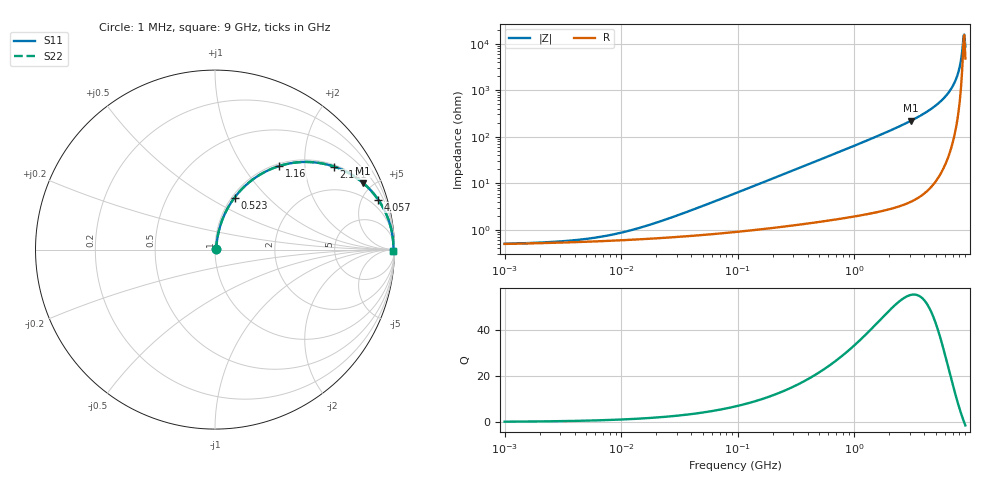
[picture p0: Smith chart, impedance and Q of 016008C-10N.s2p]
# MHz S MA R 50
!Freq  MagS11  AngS11  MagS21  AngS21  MagS12  AngS12  MagS22  AngS22
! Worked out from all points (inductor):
!   801 points, 1 MHz to 9 GHz, reference 50 ohm
!   read as one part in series: L = 10 nH near 34.45 MHz
!   highest Q = 55.1 at 3.088 GHz (marker M1), where L = 11.4 nH
!   self-resonance near 8.698 GHz
!   S11 on the Smith chart (normalised r, x): 1 MHz: 1.01, +0.00; 523 MHz: 1.03, +0.66; 1.16 GHz: 1.04, +1.48; 2.121 GHz: 1.06, +2.83; 4.057 GHz: 1.12, +6.49; 9 GHz: open
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1  0.004968 7.2  0.9951 -0.0  0.9951 -0.0  0.004968 7.2
4.59553  0.006153 27.7  0.9946 -0.2  0.9946 -0.2  0.006153 27.7
9.629812  0.008405 45.3  0.9941 -0.3  0.9941 -0.3  0.008405 45.3
20.8799  0.01458 62.7  0.9934 -0.7  0.9934 -0.7  0.01458 62.7
94.86833  0.05964 78.1  0.9894 -3.4  0.9894 -3.4  0.05964 78.1
215.2797  0.1331 77.7  0.9802 -7.6  0.9802 -7.6  0.1331 77.7
435.9703  0.2617 71.9  0.9519 -15.2  0.9519 -15.2  0.2617 71.9
523.0482  0.3094 69.4  0.937 -18.0  0.937 -18.0  0.3094 69.4
787.9209  0.4407 61.9  0.8824 -26.1  0.8824 -26.1  0.4407 61.9
1160.214  0.5883 52.4  0.7925 -36.0  0.7925 -36.0  0.5883 52.4
1980.841  0.7874 36.9  0.6002 -51.9  0.6002 -51.9  0.7874 36.9
2120.833  0.8091 34.8  0.5715 -54.0  0.5715 -54.0  0.8091 34.8
3087.586  0.9053 24.1  0.4087 -64.8  0.4087 -64.8  0.9053 24.1
4057.386  0.9506 17.0  0.2929 -71.9  0.2929 -71.9  0.9506 17.0
5580.136  0.9813 9.6  0.1664 -78.8  0.1664 -78.8  0.9813 9.6
6927.205  0.9914 4.9  0.08556 -81.8  0.08556 -81.8  0.9914 4.9
7416.771  0.993 3.5  0.06066 -81.6  0.06066 -81.6  0.993 3.5
7762.222  0.9936 2.5  0.04421 -80.5  0.04421 -80.5  0.9936 2.5
8123.764  0.994 1.6  0.02797 -76.8  0.02797 -76.8  0.994 1.6
8502.145  0.994 0.6  0.01245 -60.9  0.01245 -60.9  0.994 0.6
8797.452  0.9938 -0.1  0.006325 12.5  0.006325 12.5  0.9938 -0.1
9000  0.9936 -0.5  0.0115 55.9  0.0115 55.9  0.9936 -0.5
